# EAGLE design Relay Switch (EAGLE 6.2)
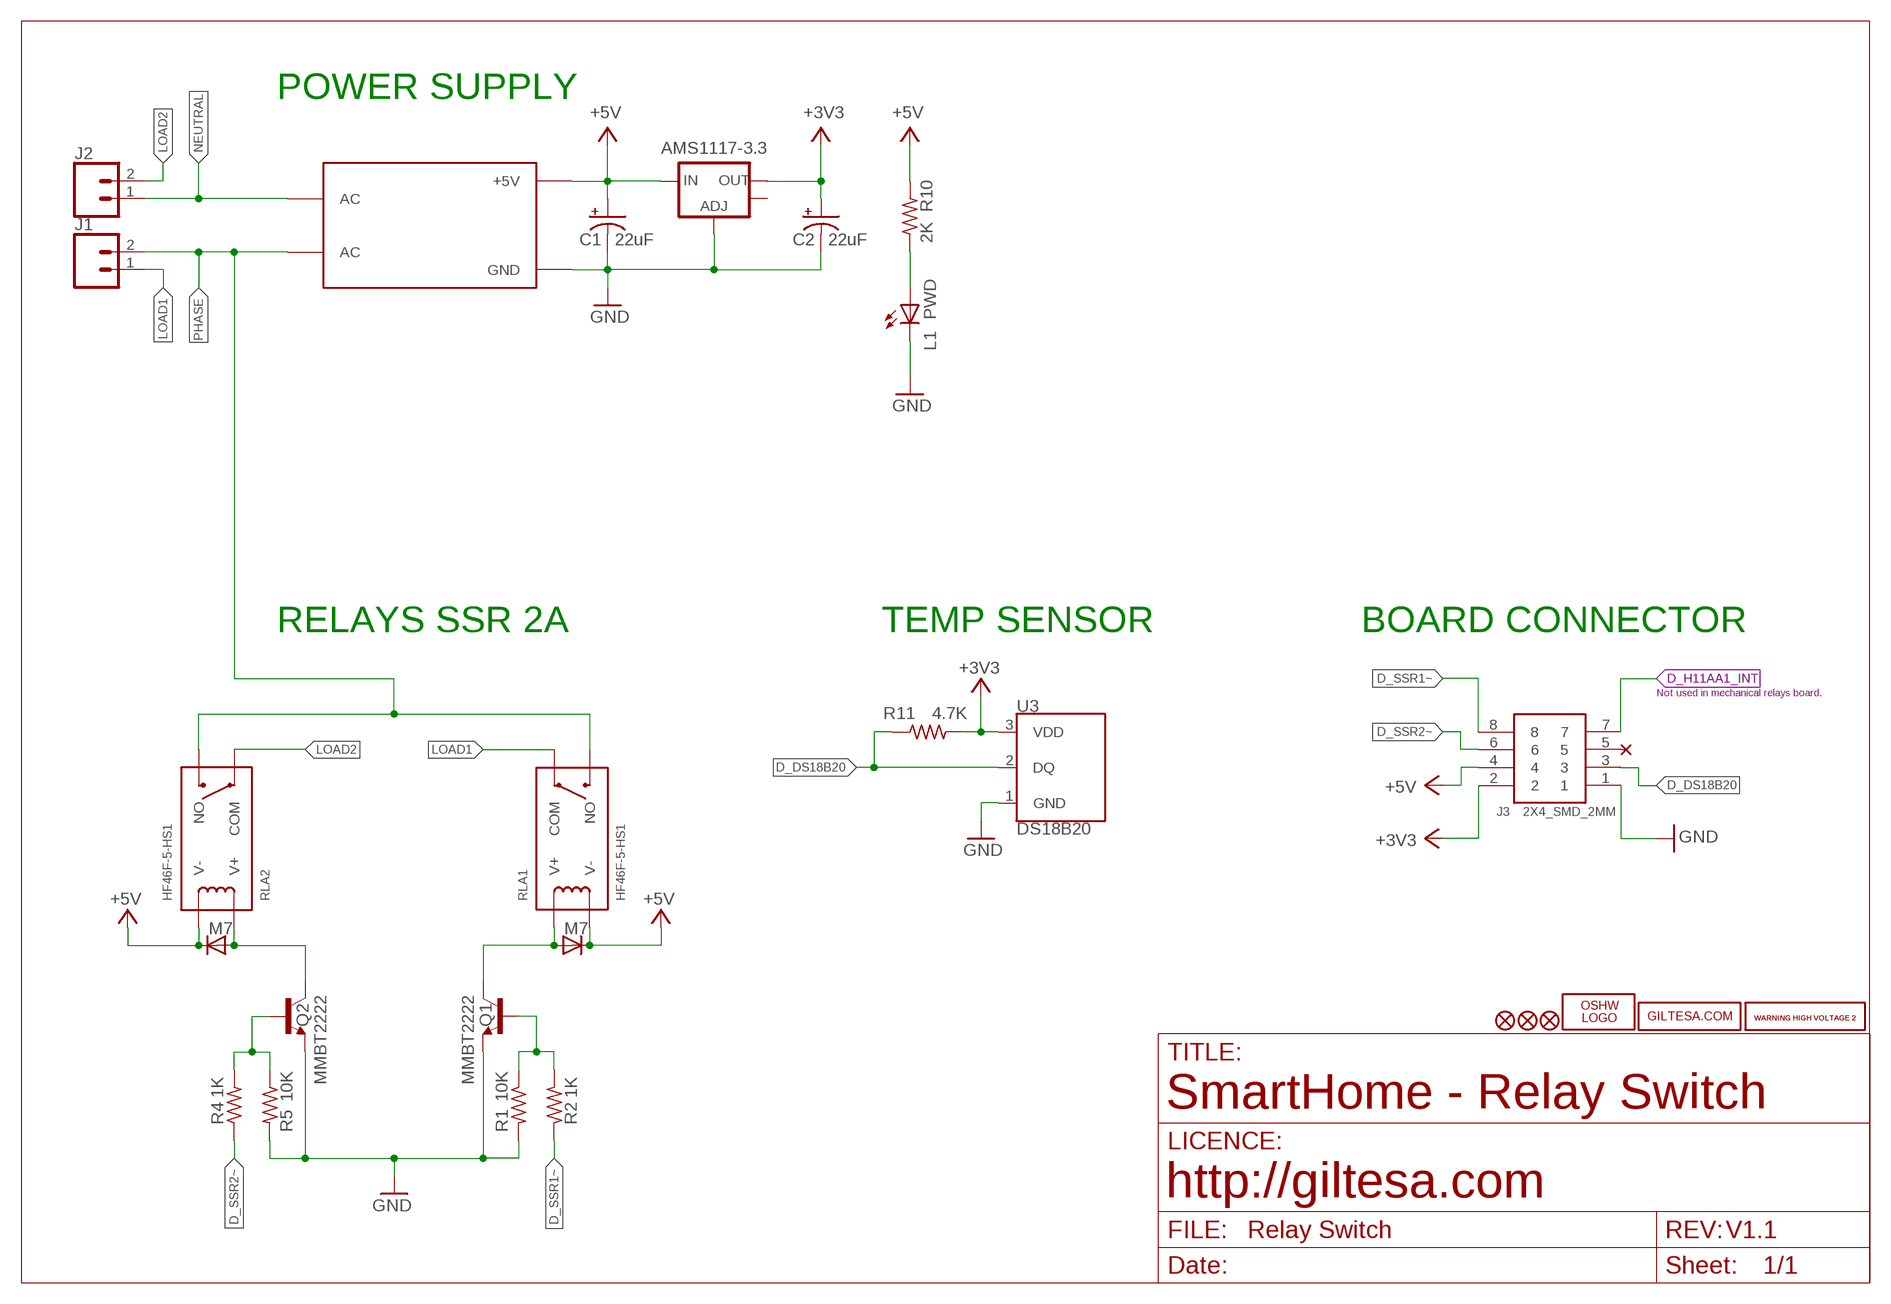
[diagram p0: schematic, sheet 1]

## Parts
AMS1117-3.3  V_REG_LM1117SOT223  [SOT223]
C1  22uF  CAP_POL3528  [EIA3528]
C2  22uF  CAP_POL3528  [EIA3528]
D1  M7  DIODE-SMB  [SMB]
D2  M7  DIODE-SMB  [SMB]
J1  TERMINAL_5MM_2P  [TERMINAL_5MM_2P]
J2  TERMINAL_5MM_2P  [TERMINAL_5MM_2P]
J3  2X4_SMD_2MM  2X4_SMD_2.0MM  [2X4_SMD_2.0MM]
L1  PWD  LEDCHIP-LED0805  [CHIP-LED0805]
LOGO1  OSHW_LOGO_FILLX0150-NT  [OSHW_FILLX150_NOTEXT]
Q1  MMBT2222  TRANSISTOR_NPNSOT23  [SOT23]
Q2  MMBT2222  TRANSISTOR_NPNSOT23  [SOT23]
R1  10K  R0603  [R0603]
R2  1K  R0603  [R0603]
R4  1K  R0603  [R0603]
R5  10K  R0603  [R0603]
R10  2K  R0603  [R0603]
R11  4.7K  R0603  [R0603]
RLA1  HF46F-5-HS1  RELAY_HF46F-5-HS1  [RELAY_HF46F-5-HS1]
RLA2  HF46F-5-HS1  RELAY_HF46F-5-HS1  [RELAY_HF46F-5-HS1]
U3  DS18B20  [DS18B20]
U$1  HILINK_HLK-PM01_5V  [HILINK_HLK-PM01_5V]
U$3  WARNING_HIGH_VOLTAGE_2  [WARNING_HIGH_VOLTAGE_2]
U$4  WARNING_HIGH_VOLTAGE_2  [WARNING_HIGH_VOLTAGE_2]
U$5  GILTESA.COM_MASK  [GILTESA.COM_MASK]
U$6  FIDUCIAL1X2  [FIDUCIAL-1X2]
U$7  FIDUCIAL1X2  [FIDUCIAL-1X2]
U$14  FIDUCIAL1X2  [FIDUCIAL-1X2]

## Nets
+3V3: AMS1117-3.3.2(OUT) C2.A(+) J3.2 R11.2 U3.3(VDD)
+5V: AMS1117-3.3.3(IN) C1.A(+) D1.C D2.C J3.4 R10.2 RLA1.V- RLA2.V- U$1.+5V
D_DS18B20: J3.3 R11.1 U3.2(DQ)
D_H11AA1_INT: J3.7
D_SSR1~: J3.8 R2.1
D_SSR2~: J3.6 R4.1
GND: AMS1117-3.3.1(ADJ) C1.C(-) C2.C(-) J3.1 L1.C Q1.2(E) Q2.2(E) R1.2 R5.2 U3.1(GND) U$1.GND
LOAD1: J1.1 RLA1.COM
LOAD2: J2.2 RLA2.COM
N$2: Q1.1(B) R1.1 R2.2
N$3: D1.A Q1.3(C) RLA1.V+
N$8: L1.A R10.1
N$46: Q2.1(B) R4.2 R5.1
N$47: D2.A Q2.3(C) RLA2.V+
NEUTRAL: J2.1 U$1.AC@2(AC)
PHASE: J1.2 RLA1.NO RLA2.NO U$1.AC@1(AC)
Unconnected: AMS1117-3.3.4(OUT) J3.5

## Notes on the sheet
- POWER SUPPLY
- RELAYS SSR 2A | TEMP SENSOR | BOARD CONNECTOR
- Not used in mechanical relays board.
- SmartHome - Relay Switch
- http://giltesa.com
- V1.1

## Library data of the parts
AMS1117-3.3 = SparkFun:V_REG_LM1117: Voltage Regulator LM1117 Standard adjustable voltage regulator but in SMD form. Spark Fun Electronics SKU : COM-00595
C1 C2 = SparkFun:CAP_POL: Capacitor Polarized
D1 D2 = diode:DIODE-: DIODE
J1 J2 = ,giltesa:TERMINAL_5MM_2P
J3 = ,giltesa:2X4_SMD_2.0MM
L1 = led:LED: LED
LOGO1 = ohw-logo:OSHW_LOGO_FILL
Q1 Q2 = SparkFun:TRANSISTOR_NPN: Transistor NPN BJT configuration in SOT23 package. MMBT2222 is the common NPN we use. Double check BCE configuration again layout.
R1 R2 R4 R5 R10 R11 = ,giltesa:R0603
RLA1 RLA2 = ,giltesa:RELAY_HF46F-5-HS1
U3 = ,giltesa:DS18B20
U$1 = ,giltesa:HILINK_HLK-PM01_5V
U$3 U$4 = ,giltesa_logos:WARNING_HIGH_VOLTAGE_2
U$5 = ,giltesa_logos:GILTESA.COM_MASK
U$6 U$7 U$14 = SparkFun:FIDUCIAL: Fiducial Alignment Points

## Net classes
0 default: width 0.203 mm

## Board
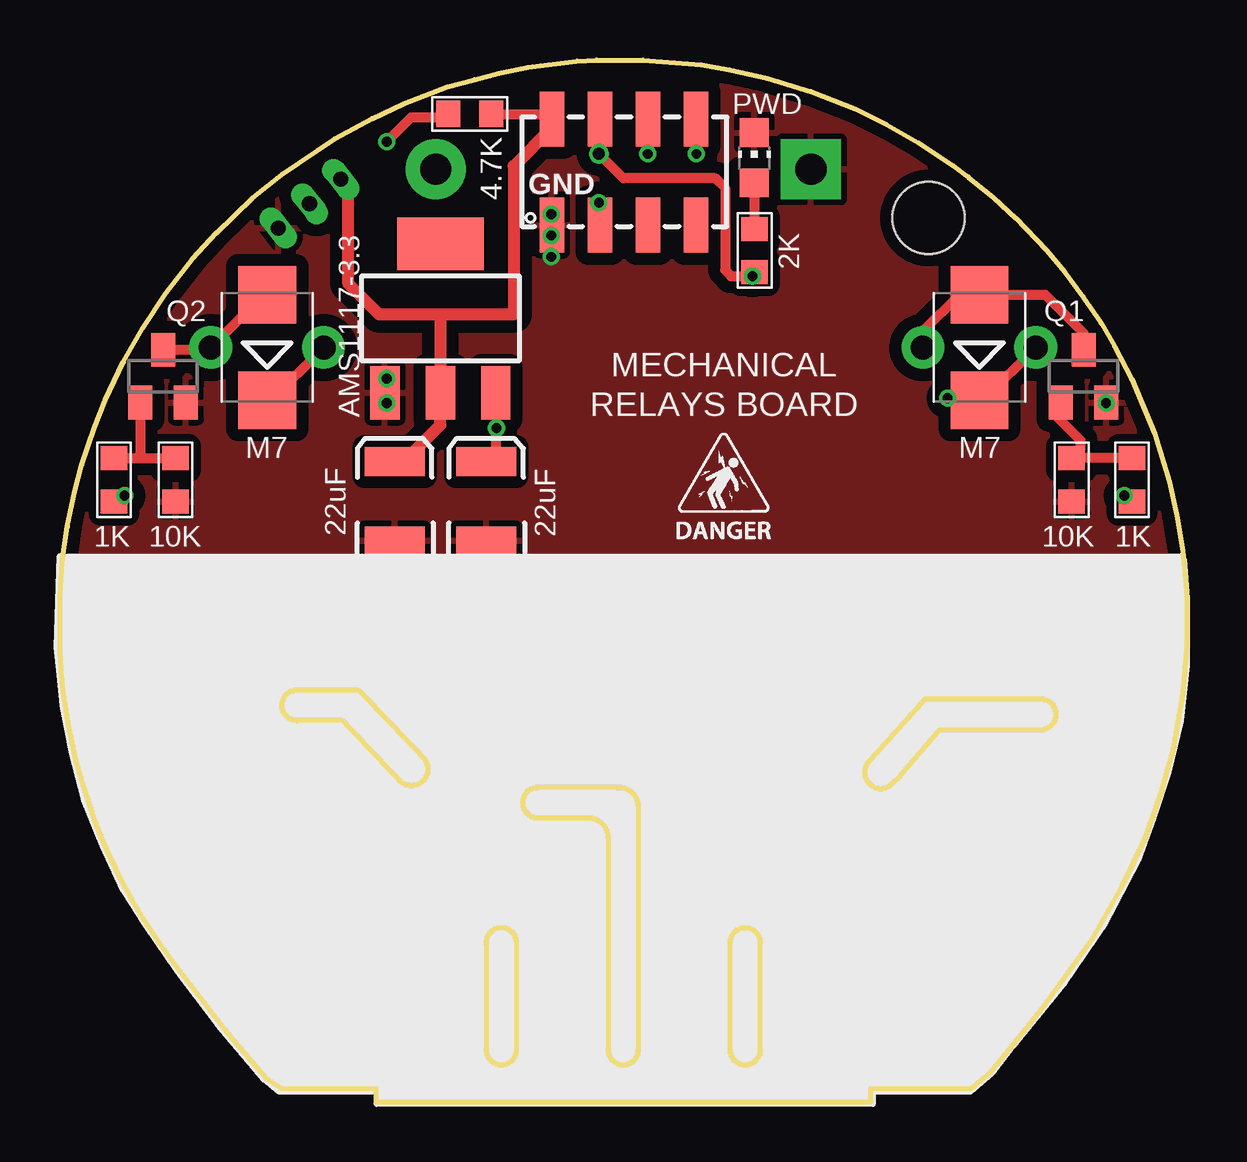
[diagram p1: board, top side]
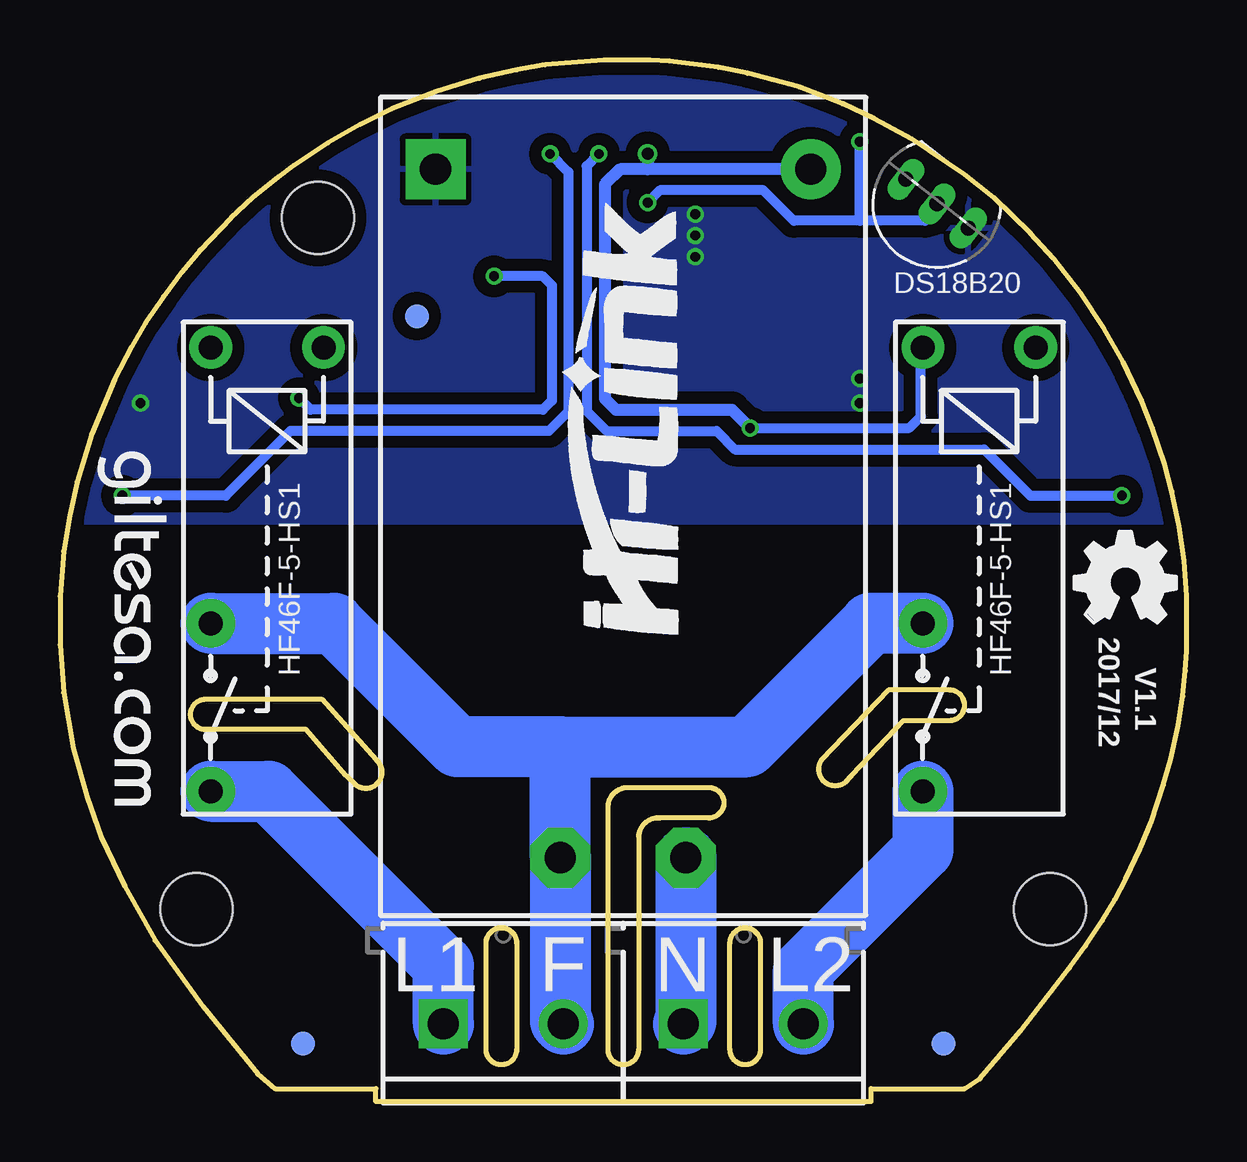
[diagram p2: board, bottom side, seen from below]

Size 46.94 x 43.43 mm. Coordinates in mm from the lower left corner, seen from the top.
Outline: 107 segments
Copper layers (1*16): Top 0.035mm / dielectric 1.6mm / Bottom 0.035mm
Design rules: minimum track width 6mil, minimum drill 12mil, track to track 6mil, track to pad 6mil, pad to pad 6mil, via to via 8mil, smd to smd 0mil, copper to edge 20mil, drill to drill 10mil, minimum pad ring 6mil, minimum via ring 6mil, stop-mask expansion 0mil, vias tented up to drill 100mil, thermal gap 10mil
Holes 3 mm at 5.69,8.03 41.25,8.03 36.19,36.84

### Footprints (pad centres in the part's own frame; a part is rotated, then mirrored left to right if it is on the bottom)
SOT223 = smd 1.219 x 2.235: 1 -2.311,-3.099; 2 0,-3.099; 3 2.311,-3.099 | smd 3.6 x 2.2: 4 0,3.099
EIA3528 = smd 1.2 x 2.5: A 1.65,0; C -1.65,0
SMB = smd 2.4 x 2.4: A 2.2,0; C -2.2,0
TERMINAL_5MM_2P = drill 1.3 pad 2.032 square: 1 0,0 | drill 1.3 pad 2.032: 2 5,0
2X4_SMD_2.0MM = smd 2.286 x 1.016: 1 -2.213,2.976; 2 2.212,2.976; 3 -2.213,0.976; 4 2.212,0.976; 5 -2.213,-1.024; 6 2.212,-1.024; 7 -2.213,-3.024; 8 2.212,-3.024
CHIP-LED0805 = smd 1.2 x 1.2: A 0,-1.05; C 0,1.05
SOT23 = smd 1 x 1.4: 1 -0.95,-1.1; 2 0.95,-1.1; 3 0,1.1
R0603 = smd 1 x 1.1: 1 -0.901,0.013; 2 0.901,0.013
RELAY_HF46F-5-HS1 = drill 1 pad 2.032: COM 9.3,-2.35; NO 2.3,-2.35 | drill 1 pad 1.778: V+ -9.2,2.35; V- -9.2,-2.35
DS18B20 = drill 0.635 pad 0.864 long: 1 -1.651,0; 2 0,0; 3 1.651,0
HILINK_HLK-PM01_5V = drill 1.3 pad 2.5: +5V 31.109,2.3 | drill 1.3 pad 2.5 octagon: AC@1 2.409,12.73; AC@2 2.409,7.5 | drill 1.3 pad 2.5 square: GND 31.109,17.93
FIDUCIAL-1X2 = smd 1 x 1: 1 0,0

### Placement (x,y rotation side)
AMS1117-3.3  15.85,32.66 0 top
C1  17.75,25.04 90 top
C2  13.94,25.04 90 top
D1  38.3,31.44 90 top
D2  8.63,31.44 90 top
J1  30.97,3.25 0 bottom
J2  20.97,3.25 0 bottom
J3  23.47,38.75 90 top
L1  28.93,39.35 0 top
LOGO1  4.67,19.96 0 bottom
Q1  42.65,30.24 0 top
Q2  4.29,30.24 0 top
R1  42.14,25.93 270 top
R2  44.68,25.93 90 top
R4  2.26,25.93 90 top
R5  4.8,25.93 270 top
R10  28.93,35.48 270 top
R11  17.07,41.16 0 top
RLA1  38.3,22.24 270 bottom
RLA2  8.63,22.24 270 bottom
U3  10.4,37.44 142 bottom
U$1  13.36,7.76 90 bottom
U$2  [ELECTROCUTION_SMALL]  25.46,23.34 0 top
U$3  0.36,12.97 0 top
U$4  43.03,12.97 0 top
U$5  45.44,27.2 270 bottom
U$6  36.8,2.43 90 bottom
U$7  10.13,2.43 90 bottom
U$14  32.07,32.74 90 bottom

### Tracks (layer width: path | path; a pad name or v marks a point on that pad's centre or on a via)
+3V3
  Top 0.406: R11.2 20.49,41.17 J3.2
  Top 0.508: C2.A 14.2,26.56 15.85,28.21 AMS1117-3.3.2 15.85,32.82 | J3.2 20.49,40.6 18.9,39.01 18.9,32.82 15.85,32.82 | 15.85,32.82 13.3,32.82 12.02,34.1 12.02,37.93 U3.3
+5V  (via drill 0.41, 0.51)
  Top 0.406: v22.45,39.51 23.47,38.5 27.31,38.5 27.71,38.1 27.71,34.67 27.97,34.41 v28.85,34.41 28.78,34.41 R10.2 | 18.19,26.81 v18.19,28.08 18.19,29.53 | D1.C 38.56,29.35 | 38.56,29.35 RLA1.V- | v36.98,29.33 38.54,29.33 38.56,29.35 | D2.C 8.78,29.24 RLA2.V-
  Top 0.508: 18.14,29.53 AMS1117-3.3.3 18.19,29.53 | J3.4 22.49,39.81 v22.45,39.51 | C1.A 18.06,26.69 18.19,26.81
  Bottom 0.406: v36.98,29.33 36.5,28.85 26.82,28.85 26.44,29.23 26.44,34.03 26.82,34.41 v28.85,34.41 | v18.19,28.08 11.56,28.08 11.07,28.57 11.07,31.35 RLA2.V-
  Bottom 0.508: U$1.+5V 22.45,38.87 | 22.45,38.87 23.6,38.87 24.23,38.24 24.23,29.3 23.77,28.85 18.95,28.85 v18.19,28.08 | v22.45,39.51 22.45,38.87
D_DS18B20  (via drill 0.41)
  Top 0.406: v22.45,37.48 22.45,36.58 J3.3 | v13.61,40.02 14.63,41.04 16.04,41.04 arc90 R11.1
  Bottom 0.406: U3.2 10.56,37.05 10.9,36.72 13.61,36.72 | 13.61,36.72 16.36,36.72 17.63,37.99 21.95,37.99 v22.45,37.48 | 13.61,36.72 v13.61,40.02
D_SSR1~  (via drill 0.41)
  Top 0.406: v26.52,39.51 26.52,40.94 J3.8 | v44.35,25.27 44.42,25.27 R2.1
  Bottom 0.406: v26.52,39.51 25.76,38.75 25.76,28.77 26.57,27.96 37.34,27.96 40.03,25.27 v44.35,25.27
D_SSR2~  (via drill 0.41)
  Top 0.406: v24.49,39.51 J3.6 | v2.69,25.27 2.49,25.27 R4.1
  Bottom 0.406: v24.49,39.51 24.99,39.01 24.99,28.8 24.16,27.96 19.58,27.96 18.82,27.2 8.43,27.2 6.5,25.27 v2.69,25.27
GND  (via drill 0.41)
  other vias: 43.59,29.13 13.61,30.14 13.61,29.13 20.47,37 20.47,36.11 20.47,35.22
  pour Top (isolate 0.508): -0.03,22.88 46.96,22.88 46.96,23.77 46.33,26.31 45.06,29.48 42.52,33.93 39.98,37.1 35.53,40.28 29.82,42.82 24.74,43.45 20.93,43.45 15.85,42.18 10.77,39.64 6.96,36.47 3.78,32.66 1.88,29.48 -0.03,23.77
  pour Bottom (isolate 0.508): -0.03,24.15 46.96,24.15 46.33,26.31 45.06,29.48 42.52,33.93 39.98,37.1 35.53,40.28 29.82,42.82 24.74,43.45 20.93,43.45 15.85,42.18 10.77,39.64 6.96,36.47 3.78,32.66 1.88,29.48
LOAD1
  Bottom 2.54: J1.1 30.97,5.67 38.25,12.94 RLA1.COM
LOAD2
  Bottom 2.54: J2.2 15.97,5.52 10.98,10.5 RLA2.COM
N$2
  Top 0.406: R2.2 R1.1 42.52,27.22 42.52,27.58 41.44,28.65 Q1.1
N$3
  Top 0.406: Q1.3 42.65,32.05 41.06,33.64 D1.A 38.55,33.65 37.49,33.65 35.95,32.11 RLA1.V+
N$8
  Top 0.406: R10.1 28.94,38.29 L1.A
N$46
  Top 0.406: R4.2 3.2,26.83 | 3.2,26.83 R5.1 | Q2.1 3.34,26.97 3.2,26.83
N$47
  Top 0.406: D2.A 8.38,33.54 RLA2.V+ 6.19,31.34 Q2.3
NEUTRAL
  Bottom 2.54: U$1.AC@2 20.86,3.35 J2.1
PHASE
  Bottom 2.54: 26.09,14.8 U$1.AC@1 26.09,3.37 J1.2 | 26.09,14.8 18.31,14.8 13.17,19.94 RLA2.NO | 26.09,14.8 30.38,14.8 35.53,19.94 RLA1.NO

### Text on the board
tPlace: GND | MECHANICAL | RELAYS BOARD
bPlace: 2017/12 | V1.1 | L2 | N | F | L1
